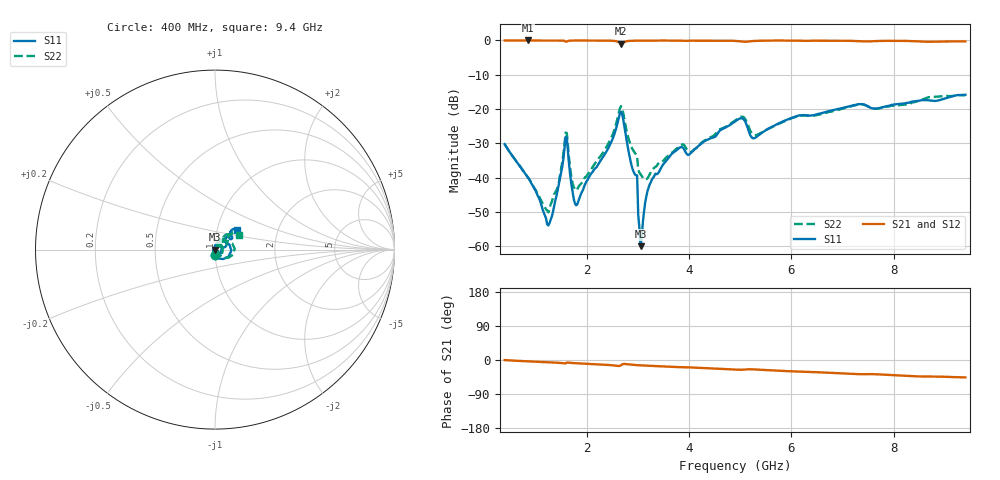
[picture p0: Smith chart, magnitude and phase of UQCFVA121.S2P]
!  Part Number  UQCFVA121  Mounting Orientation: Horizontal
!  Description: Ultra Low ESR Microwave capacitors
!  Application: Coupling, Bypass, Tuning, DC Block
!  Filters, Matching
# GHZ S DB R 50
! Freq  |S11|  S11 Ph  |S21|  S21 Ph  |S12|  S12 Ph  |S22|  S22 Ph
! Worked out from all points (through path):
!   401 points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, 400 MHz to 9.4 GHz, reference 50 ohm
!   highest |S21| = -0.01 dB at 850 MHz (marker M1); lowest = -0.9 dB at 2.673 GHz (marker M2)
!   group delay of S21, straight-line fit = 14.1 ps
!   lowest |S11| = -59.9 dB at 3.055 GHz (marker M3), VSWR 1.00, Z = 49.9 - j0.032 ohm
!   |S11| at or under -10 dB: start of sweep to end of sweep
!   |S22| runs from -50.1 to -15.9 dB; largest |S21 - S12| = 0.0033
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0.4  -30.19 -89.3  -0.02 -0.2  -0.02 -0.2  -30.19 -88.0
0.85  -39.89 -97.2  -0.01 -3.5  -0.02 -3.5  -39.75 -81.8
1.278  -53.15 168.4  -0.02 -6.2  -0.02 -6.2  -48.93 6.7
1.458  -42.02 94.2  -0.03 -7.4  -0.03 -7.4  -41.54 50.5
1.593  -28.04 20.6  -0.35 -8.8  -0.35 -8.7  -26.82 17.6
1.638  -32.32 -63.2  -0.17 -6.7  -0.17 -6.7  -30.86 -47.4
1.773  -47.43 -160.4  -0.03 -8.4  -0.03 -8.3  -43.35 -16.6
1.908  -44.20 128.2  -0.03 -9.3  -0.02 -9.3  -41.45 25.7
2.403  -31.99 84.5  -0.06 -12.8  -0.06 -12.8  -30.67 53.1
2.673  -20.80 -3.1  -0.94 -13.9  -0.93 -13.9  -19.16 2.7
2.943  -38.92 -160.4  -0.08 -13.2  -0.08 -13.2  -32.74 -32.4
3.055  -59.91 -161.5  -0.06 -14.1  -0.06 -14.1  -38.97 -21.6
3.213  -42.82 84.8  -0.05 -15.2  -0.05 -15.2  -39.59 24.6
3.415  -38.31 77.3  -0.04 -16.4  -0.04 -16.4  -35.63 41.6
3.798  -31.42 62.4  -0.07 -18.8  -0.07 -18.8  -31.00 49.5
4.023  -33.01 60.6  -0.08 -19.5  -0.08 -19.5  -32.50 46.1
4.9  -23.61 49.9  -0.13 -25.1  -0.14 -25.1  -23.37 54.2
5.058  -22.81 27.3  -0.36 -25.6  -0.36 -25.6  -22.25 34.7
5.283  -28.47 36.2  -0.15 -24.9  -0.15 -24.9  -27.57 36.4
6.408  -21.83 45.4  -0.09 -31.7  -0.10 -31.7  -21.96 53.6
7.915  -18.97 43.0  -0.11 -39.4  -0.11 -39.4  -19.19 45.5
9.4  -15.81 41.3  -0.27 -46.0  -0.27 -46.0  -15.97 31.0
